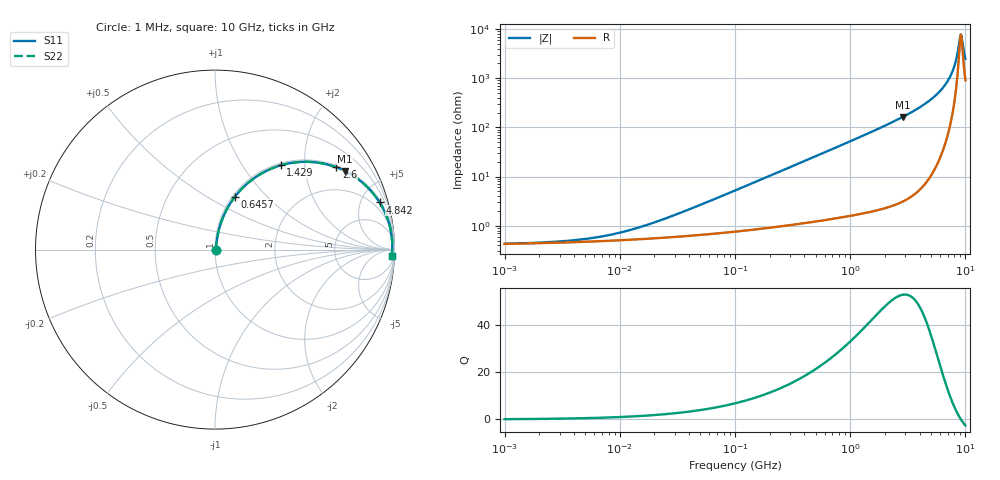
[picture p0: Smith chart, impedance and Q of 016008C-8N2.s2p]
# MHz S MA R 50
!Freq  MagS11  AngS11  MagS21  AngS21  MagS12  AngS12  MagS22  AngS22
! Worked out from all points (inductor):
!   801 points, 1 MHz to 10 GHz, reference 50 ohm
!   read as one part in series: L = 8.2 nH near 35.48 MHz
!   highest Q = 52.6 at 2.851 GHz (marker M1), where L = 9.08 nH
!   self-resonance near 9.12 GHz
!   S11 on the Smith chart (normalised r, x): 1 MHz: 1.01, +0.00; 645.7 MHz: 1.03, +0.67; 1.429 GHz: 1.04, +1.51; 2.6 GHz: 1.06, +2.92; 4.842 GHz: 1.18, +6.93; 10 GHz: 19, -46
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1  0.004281 6.9  0.9958 -0.0  0.9958 -0.0  0.004281 6.9
4.677351  0.005253 27.0  0.9953 -0.1  0.9953 -0.1  0.005253 27.0
9.885531  0.007141 44.9  0.995 -0.3  0.995 -0.3  0.007141 44.9
21.62719  0.01241 62.6  0.9944 -0.6  0.9944 -0.6  0.01241 62.6
101.1579  0.05221 78.7  0.9911 -3.0  0.9911 -3.0  0.05221 78.7
231.7395  0.1179 78.7  0.9837 -6.7  0.9837 -6.7  0.1179 78.7
467.7351  0.2325 73.8  0.9612 -13.4  0.9612 -13.4  0.2325 73.8
645.6542  0.3136 69.5  0.9371 -18.3  0.9371 -18.3  0.3136 69.5
966.0509  0.4443 61.9  0.8822 -26.4  0.8822 -26.4  0.4443 61.9
1428.894  0.5954 52.1  0.7888 -36.5  0.7888 -36.5  0.5954 52.1
2162.719  0.7555 39.8  0.64 -49.1  0.64 -49.1  0.7555 39.8
2600.16  0.8173 34.1  0.5606 -54.8  0.5606 -54.8  0.8173 34.1
2851.018  0.8449 31.3  0.5191 -57.6  0.5191 -57.6  0.8449 31.3
4841.724  0.9542 16.0  0.2752 -72.5  0.2752 -72.5  0.9542 16.0
6095.369  0.9771 10.0  0.173 -77.4  0.173 -77.4  0.9771 10.0
7244.36  0.9859 5.6  0.0988 -79.0  0.0988 -79.0  0.9859 5.6
8035.261  0.988 3.1  0.05548 -76.0  0.05548 -76.0  0.988 3.1
8317.638  0.9882 2.3  0.04143 -72.3  0.04143 -72.3  0.9882 2.3
8810.489  0.9879 0.9  0.01983 -51.9  0.01983 -51.9  0.9879 0.9
9015.711  0.9876 0.4  0.01386 -26.1  0.01386 -26.1  0.9876 0.4
9332.543  0.9869 -0.5  0.01548 31.7  0.01548 31.7  0.9869 -0.5
10000  0.9847 -2.1  0.03982 66.3  0.03982 66.3  0.9847 -2.1
